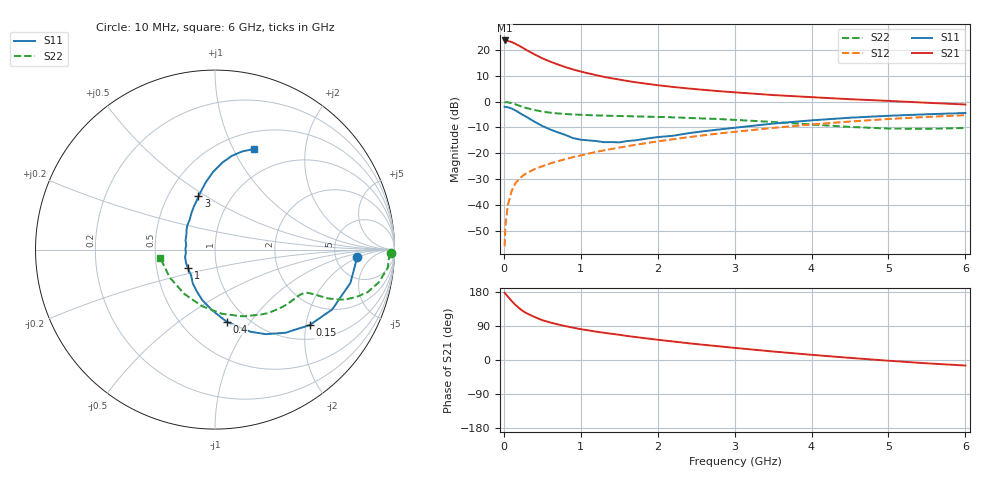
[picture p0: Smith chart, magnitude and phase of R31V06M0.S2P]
! SIEMENS Small Signal Semiconductors
! BFR181
! Si NPN RF Bipolar Junction Transistor in SOT23
! VCE = 1 V  IC = 6 mA
! Common Emitter S-Parameters:  May  1996
# GHz  S  MA  R  50
!  f  S11  S21  S12  S22
! GHz  MAG  ANG  MAG  ANG  MAG  ANG  MAG  ANG
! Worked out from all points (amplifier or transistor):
!   36 points, 10 MHz to 6 GHz, reference 50 ohm
!   highest |S21| = 23.6 dB at 10 MHz (marker M1)
!   |S21| within 3 dB of that: start of sweep to 255.2 MHz
!   unconditionally stable (mu >= 1): 791.8 MHz to 3.139 GHz
!   at 250 MHz: K = 0.51, MSG = 24.6 dB, |S12| = -28.6 dB
!   at 1.4 GHz: K = 1.11, MAG = 11.6 dB, |S12| = -18.4 dB
!   at 6 GHz: K = 0.90, MSG = 2.1 dB, |S12| = -5.3 dB
!   S11 on the Smith chart (normalised r, x): 10 MHz: 8.13, -1.79; 150 MHz: 1.36, -2.10; 400 MHz: 0.81, -0.77; 1 GHz: 0.72, -0.16; 3 GHz: 0.71, +0.46; 6 GHz: 0.69, +1.20
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0.01  0.7902 -3.0  15.15 177.5  0.0016 89.4  0.9801 -1.2
0.02  0.7871 -5.5  14.93 174.9  0.0039 87.9  0.9711 -2.4
0.05  0.777 -13.8  14.84 167.8  0.0096 82.4  0.9676 -6.0
0.1  0.733 -27.1  14.18 156.1  0.0185 75.8  0.9308 -11.3
0.15  0.6744 -38.6  13.02 145.4  0.0263 71.2  0.8827 -15.6
0.2  0.6075 -49.7  11.96 136.6  0.032 67.6  0.8311 -18.5
0.25  0.5497 -59.0  10.84 128.8  0.0372 64.5  0.7835 -20.7
0.3  0.498 -66.7  9.79 123.0  0.0416 63.9  0.7426 -22.0
0.4  0.4066 -80.9  8.143 113.4  0.0495 61.7  0.6843 -23.4
0.5  0.3371 -93.0  6.836 105.1  0.0562 61.8  0.6399 -23.9
0.6  0.2896 -104.3  5.931 99.1  0.0634 61.7  0.6088 -24.2
0.8  0.2259 -123.1  4.631 89.4  0.0771 62.8  0.5742 -24.9
1  0.183 -145.4  3.799 81.4  0.0911 63.6  0.5536 -26.0
1.1  0.1773 -155.5  3.498 78.2  0.0986 64.3  0.546 -26.7
1.3  0.1637 -172.9  2.998 72.0  0.1136 64.4  0.5344 -28.4
1.6  0.1721 162.5  2.503 63.5  0.137 64.1  0.5215 -31.6
2.2  0.218 130.4  1.913 48.9  0.1868 62.0  0.4942 -40.1
3  0.311 107.2  1.506 32.0  0.2597 56.4  0.4425 -54.9
3.5  0.3747 98.3  1.334 22.4  0.3092 51.9  0.4025 -67.5
4.5  0.4863 85.2  1.11 5.6  0.4108 40.4  0.3227 -103.1
5.5  0.5671 74.6  0.946 -8.8  0.5046 27.0  0.2963 -148.3
6  0.6001 69.0  0.876 -14.6  0.5447 19.6  0.3081 -170.9
